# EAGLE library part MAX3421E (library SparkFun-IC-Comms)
MAX3421EEHJ USB Peripheral / Host Controller. SPI, 32TQFP SparkFun Products SparkFun USB Host Shield (DEV-09947)
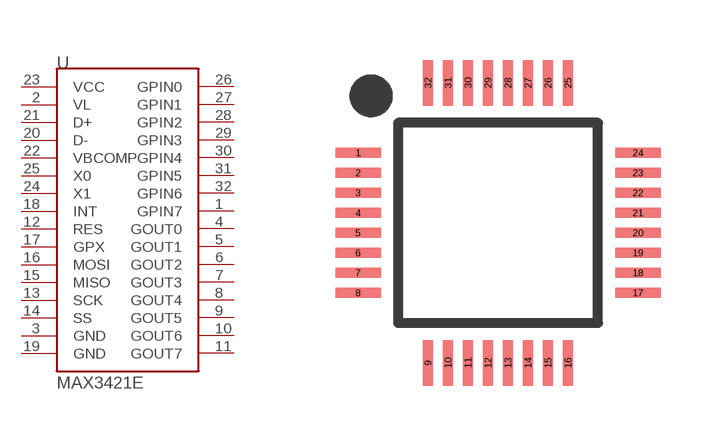
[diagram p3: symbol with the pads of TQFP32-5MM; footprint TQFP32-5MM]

Designator prefix U

## MAX3421ESMD (PROD_ID: IC-09517; VALUE: MAX3421)  [TQFP32-5MM]
1  GPIN7
2  VL
3  GND
4  GOUT0
5  GOUT1
6  GOUT2
7  GOUT3
8  GOUT4
9  GOUT5
10  GOUT6
11  GOUT7
12  RES
13  SCK
14  SS
15  MISO
16  MOSI
17  GPX
18  INT
19  GND
20  D-
21  D+
22  VBCOMP
23  VCC
24  X1
25  X0
26  GPIN0
27  GPIN1
28  GPIN2
29  GPIN3
30  GPIN4
31  GPIN5
32  GPIN6

## Footprint TQFP32-5MM (pad centres in mm)
TQFP - 32 Specifications: Pin count: 32 Pin pitch:5mm Example device(s): MAX3421E
smd 1.143 x 0.254: 1 -3.5,1.75; 2 -3.5,1.25; 3 -3.5,0.75; 4 -3.5,0.25; 5 -3.5,-0.25; 6 -3.5,-0.75; 7 -3.5,-1.25; 8 -3.5,-1.75; 17 3.5,-1.75; 18 3.5,-1.25; 19 3.5,-0.75; 20 3.5,-0.25; 21 3.5,0.25; 22 3.5,0.75; 23 3.5,1.25; 24 3.5,1.75
smd 0.254 x 1.143: 9 -1.75,-3.5; 10 -1.25,-3.5; 11 -0.75,-3.5; 12 -0.25,-3.5; 13 0.25,-3.5; 14 0.75,-3.5; 15 1.25,-3.5; 16 1.75,-3.5; 25 1.75,3.5; 26 1.25,3.5; 27 0.75,3.5; 28 0.25,3.5; 29 -0.25,3.5; 30 -0.75,3.5; 31 -1.25,3.5; 32 -1.75,3.5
